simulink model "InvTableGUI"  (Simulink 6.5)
settings: Solver=FixedStepDiscrete  StartTime=0.0  StopTime=inf  FixedStep=samplePeriod  RelTol=1e-3
PreLoadFcn:
  | initialize
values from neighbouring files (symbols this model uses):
  accelCanon = 9810    [initialize.m]
  aInv = bFwd / bFwd(1)    [initialize.m]
  bInv = aFwd / bFwd(1)    [initialize.m]
  flowCanon = 1.666667e+04    (= 16666.67)    [initialize.m]    (also in Copy of initialize.m)
  forceCanon = 1    [initialize.m]    (also in Copy of initialize.m)
  friction = 5			 				* 0.155000	 				* 0.00444822 				* area1    (= 2.71252900422)    [initialize.m]
  gasConstant = 1.8    [initialize.m]    (also in Copy of initialize.m)
  iactParams = [actParams, dfGain, solver]    [initialize.m]
  lengthCanon = 1    [initialize.m]    (also in Copy of initialize.m)
  massCanon = 1e-06    [initialize.m]    (also in Copy of initialize.m)
  maxOilVolume = volume * (1 - (precharge/supplyPress)^(1/gasConstant))    (= 211.391477114)    [initialize.m]    (also in Copy of initialize.m)
  precharge = 3000		 				* 6.894757e-03    (= 20.684271)    [initialize.m]    (also in Copy of initialize.m)
  pumpFlow = 1e20    (= 1e+20)    [initialize.m]    (also in Copy of initialize.m)
  returnPress = 3			 				* 0.1    (= 0.3)    [initialize.m]    (also in Copy of initialize.m)
  rigidMass = 32900		 				+ (   3596	 				   +   528	 				   +    43	 				   +   122)	 				* 0.453592    (= 34845.456088)    [initialize.m]
  samplePeriod = controlPeriod/upsampleFactor    (= 0.0009765625)    [initialize.m]    (also in viewer.m = eval(getHeaderValue(header, 'DELTA_T')); Copy of initialize.m)
  supplyPress = 280		 				* 0.1    (= 28)    [initialize.m]    (also in Copy of initialize.m)
  velocCanon = 1    [initialize.m]    (also in Copy of initialize.m)
  volume = 15.15		 				+ (  45		 				    * 2		 				   + 30		 				    * 6 )	 				* 5    (= 1365.15)    [initialize.m]    (also in quake.m = volume / 231.0; Copy of initialize.m)
  volumeCanon = 1e+06    (= 1000000)    [initialize.m]    (also in Copy of initialize.m)
  yieldDispl = 1.0    (= 1)    [initialize.m]
undefined symbols (not defined in the file or in its folder): DiscIntNeverNeededParam
libraries: simulink x1

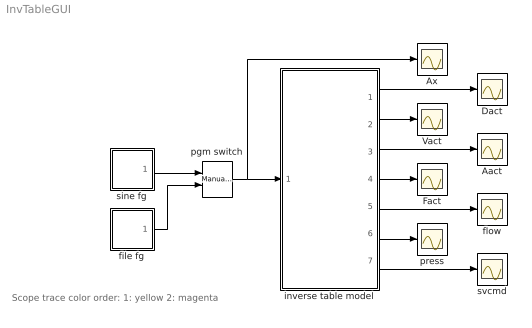
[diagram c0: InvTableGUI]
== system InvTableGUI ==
  note: Scope trace color order: 1: yellow 2: magenta
  Aact : Scope
  Ax : Scope
  Dact : Scope
  Fact : Scope
  Vact : Scope
  file fg : Subsystem
  flow : Scope
  inverse table model : Subsystem
  pgm switch : simulink/Signal Routing/Manual Switch  SystemSampleTime=-1  sw=1  action=0
  press : Scope
  sine fg : Subsystem  mask(Sine Function Generator){ampl=0.5, freq=0.5, spanInterval=1, samplePeriod=samplePeriod}
      mask prompts: ampl "Amplitude"; freq "Frequency (Hz)"; spanInterval "Span interval (sec)"; samplePeriod "Sample period (sec)"
  svcmd : Scope
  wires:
  sine fg/1(out) -> pgm switch/1
  pgm switch/1 -> Ax/1, inverse table model/1(Ax)
  inverse table model/1(Dact) -> Dact/1
  inverse table model/2(Vact) -> Vact/1
  inverse table model/3(Aact) -> Aact/1
  inverse table model/4(Fact) -> Fact/1
  inverse table model/5(flow) -> flow/1
  inverse table model/6(press) -> press/1
  inverse table model/7(svcmd) -> svcmd/1
  file fg/1(out) -> pgm switch/2

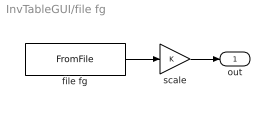
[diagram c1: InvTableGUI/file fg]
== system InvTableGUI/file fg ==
  file fg : FromFile  FileName=KobeAccel.mat  SampleTime=samplePeriod
  scale : Gain
  out : Outport
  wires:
  scale/1 -> out/1
  file fg/1 -> scale/1

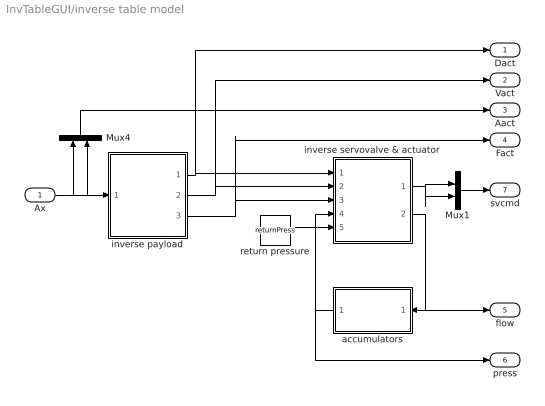
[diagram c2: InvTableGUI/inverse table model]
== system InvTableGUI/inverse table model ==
  Ax : Inport
  Mux1 : Mux  Inputs=2
  Mux4 : Mux  Orientation=up  Inputs=2
  accumulators : Subsystem  Orientation=left
  inverse payload : Subsystem
  inverse servovalve & actuator : Subsystem  mask(Inverse actuator){params=iactParams}
      mask prompts: params "Parameter vector"
  return pressure : Constant  Value=returnPress  OutDataType=sfix(16)  ConRadixGroup=Use specified scaling  OutScaling=2^0  SampleTime=inf  FramePeriod=inf
  Dact : Outport
  Vact : Outport  Port=2
  Aact : Outport  Port=3
  Fact : Outport  Port=4
  flow : Outport  Port=5
  press : Outport  Port=6
  svcmd : Outport  Port=7
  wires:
  inverse payload/3(force) -> inverse servovalve & actuator/3(force), Fact/1
  inverse payload/2(veloc) -> inverse servovalve & actuator/2(veloc), Vact/1
  inverse payload/1(displ) -> inverse servovalve & actuator/1(displ), Dact/1
  Mux1/1 -> svcmd/1
  inverse servovalve & actuator/1(cmd) -> Mux1/2, Mux1/1
  inverse servovalve & actuator/2(flow) -> flow/1, accumulators/1(flow)
  return pressure/1 -> inverse servovalve & actuator/5(rtn press)
  accumulators/1(press) -> inverse servovalve & actuator/4(spl press), press/1
  Mux4/1 -> Aact/1
  Ax/1 -> Mux4/2, inverse payload/1(accel), Mux4/1

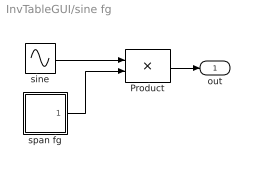
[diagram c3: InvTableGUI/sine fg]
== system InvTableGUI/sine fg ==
  Product : Product
  sine : Sin  Amplitude=ampl  Frequency=2 * pi * freq  SampleTime=samplePeriod
  span fg : Subsystem  mask{spanInterval=spanInterval, samplePeriod=samplePeriod}
      mask prompts: spanInterval "Span interval (sec)"; samplePeriod "Sample period (sec)"
  out : Outport
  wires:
  span fg/1(out) -> Product/2
  sine/1 -> Product/1
  Product/1 -> out/1

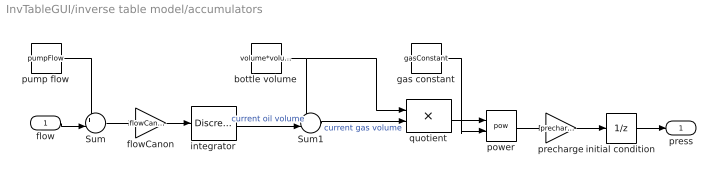
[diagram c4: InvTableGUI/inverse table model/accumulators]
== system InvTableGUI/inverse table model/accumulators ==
  flow : Inport
  Sum : Sum  Inputs=+-|
  Sum1 : Sum  Inputs=+-|
  bottle volume : Constant  Value=volume*volumeCanon  OutDataType=sfix(16)  ConRadixGroup=Use specified scaling  OutScaling=2^0  SampleTime=inf  FramePeriod=inf
  flowCanon : Gain  Gain=flowCanon
  gas constant : Constant  Value=gasConstant  OutDataType=sfix(16)  ConRadixGroup=Use specified scaling  OutScaling=2^0  SampleTime=inf  FramePeriod=inf
  initial condition : UnitDelay  X0=supplyPress  SampleTime=-1
  integrator : DiscreteIntegrator  InitialCondition=maxOilVolume*volumeCanon  SampleTime=-1  LimitOutput=on  UpperSaturationLimit=maxOilVolume*volumeCanon  LowerSaturationLimit=0  ICPrevOutput=DiscIntNeverNeededParam  ICPrevScaledInput=DiscIntNeverNeededParam
  power : Math  Operator=pow
  precharge : Gain  Gain=precharge
  pump flow : Constant  Value=pumpFlow  OutDataType=sfix(16)  ConRadixGroup=Use specified scaling  OutScaling=2^0  SampleTime=inf  FramePeriod=inf
  quotient : Product  Inputs=*/
  press : Outport
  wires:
  initial condition/1 -> press/1
  flowCanon/1 -> integrator/1
  flow/1 -> Sum/2
  integrator/1 -> Sum1/2  "current oil volume"
  quotient/1 -> power/1
  Sum1/1 -> quotient/2  "current gas volume"
  precharge/1 -> initial condition/1
  power/1 -> precharge/1
  gas constant/1 -> power/2
  bottle volume/1 -> quotient/1, Sum1/1
  Sum/1 -> flowCanon/1
  pump flow/1 -> Sum/1

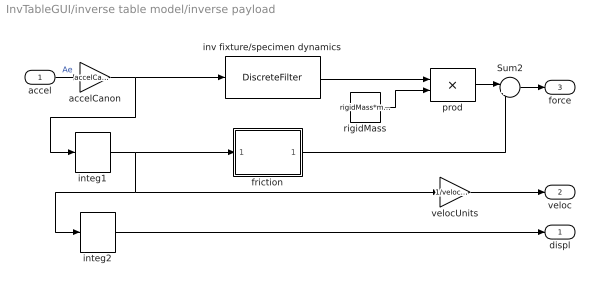
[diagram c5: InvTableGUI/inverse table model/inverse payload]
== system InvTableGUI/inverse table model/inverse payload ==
  accel : Inport
  Sum2 : Sum  Inputs=|++
  accelCanon : Gain  Gain=accelCanon
  friction : Subsystem  mask{friction=friction*forceCanon, yieldDispl=yieldDispl*lengthCanon, hysteresis=0}
      mask prompts: friction "Sliding friction"; yieldDispl "Equiv. yield displacement (in)"; hysteresis "Hysteresis constant"
  integ1 : DiscreteIntegrator  IntegratorMethod=Integration: Backward Euler  SampleTime=-1  ICPrevOutput=DiscIntNeverNeededParam  ICPrevScaledInput=DiscIntNeverNeededParam
  integ2 : DiscreteIntegrator  IntegratorMethod=Integration: Backward Euler  SampleTime=-1  ICPrevOutput=DiscIntNeverNeededParam  ICPrevScaledInput=DiscIntNeverNeededParam
  inv fixture/specimen dynamics : DiscreteFilter  Numerator=bInv  Denominator=aInv  SampleTime=-1
  prod : Product  Inputs=**
  rigidMass : Constant  Value=rigidMass*massCanon  OutDataType=sfix(16)  ConRadixGroup=Use specified scaling  OutScaling=2^0  SampleTime=inf  FramePeriod=inf
  velocUnits : Gain  Gain=1/velocCanon
  displ : Outport
  veloc : Outport  Port=2
  force : Outport  Port=3
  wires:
  velocUnits/1 -> veloc/1
  Sum2/1 -> force/1
  accel/1 -> accelCanon/1  "Ae"
  accelCanon/1 -> inv fixture/specimen dynamics/1, integ1/1
  integ1/1 -> velocUnits/1, integ2/1, friction/1(veloc)
  integ2/1 -> displ/1
  friction/1(force) -> Sum2/2
  inv fixture/specimen dynamics/1 -> prod/1
  prod/1 -> Sum2/1
  rigidMass/1 -> prod/2

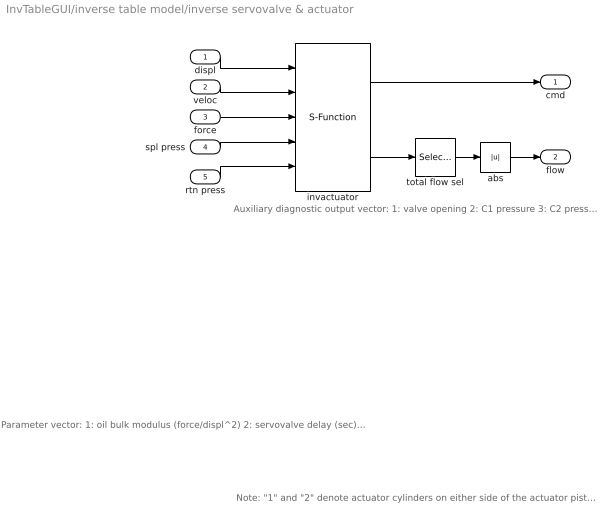
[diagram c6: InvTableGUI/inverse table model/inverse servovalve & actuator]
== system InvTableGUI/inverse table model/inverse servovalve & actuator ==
  note: Auxiliary diagnostic output vector: 1: valve opening 2: C1 pressure 3: C2 pressure 4: delta pressure 5: force 6: velocity 7: C1 flow 8: C2 flow 9: total flow 10: kinematic flow 11: compressibility flow 12: leakage flow 13: C1 oilspring displacement 14: C2 oilspring displacement 15: C1 oilspring velocity 16: C2 oilspring velocity 17: iteration error
  note: Note: "1" and "2" denote actuator cylinders on either side of the actuator piston. With positive valve drive, oil is ported into cylinder 1, resulting in positive displacement.
  note: Parameter vector: 1: oil bulk modulus (force/displ^2) 2: servovalve delay (sec) 3: servovalve overlap 4: rated pressure (force/displ^2) 5: rated flow at rated pressure (displ^3/sec) 6: nominal flow at rated pressure (displ^3/sec) 7: actuator piston area 1 (displ^2) 8: actuator piston area 2 (displ^2) 9: actuator usable stroke 1 (displ) 10: actuator usable stroke 2 (displ) 11: actuator end cushion length 1 (displ) 12: actuator end cushion length 2 (displ) 13: additional port volume 1 (displ^3) 14: additional port volume 1 (displ^3) 15: actuator parasitic damping factor 16: cross-chamber leakage factor (flow/press) 17: ratio port openings according to area 18: sample period (sec) Conversion factors used for converting signals from external (user) to internal (canonical) units: 19: displacement 20: velocity 21: force 22: pressure 23: flow Other: 24: delta-F feedback gain 25: inverse solver (0: exact, 1: approx)
  displ : Inport
  veloc : Inport  Port=2
  force : Inport  Port=3
  spl press : Inport  Port=4
  rtn press : Inport  Port=5
  abs : Abs  SaturateOnIntegerOverflow=on  SampleTime=-1
  invactuator : S-Function  FunctionName=InvActuator  Parameters=params
  total flow sel : Selector  InputType=Vector  ElementSrc=Internal  Elements=9  RowSrc=Internal  Rows=1  ColumnSrc=Internal  Columns=1  IndexIsStartValue=off
  cmd : Outport
  flow : Outport  Port=2
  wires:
  abs/1 -> flow/1
  total flow sel/1 -> abs/1
  invactuator/2 -> total flow sel/1
  force/1 -> invactuator/3
  veloc/1 -> invactuator/2
  invactuator/1 -> cmd/1
  displ/1 -> invactuator/1
  rtn press/1 -> invactuator/5
  spl press/1 -> invactuator/4

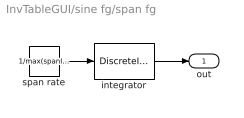
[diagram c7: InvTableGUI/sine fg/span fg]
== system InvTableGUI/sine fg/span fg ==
  integrator : DiscreteIntegrator  SampleTime=samplePeriod  LimitOutput=on  UpperSaturationLimit=1  LowerSaturationLimit=0  ICPrevOutput=DiscIntNeverNeededParam  ICPrevScaledInput=DiscIntNeverNeededParam
  span rate : Constant  Value=1/max(spanInterval,samplePeriod)  OutDataType=sfix(16)  ConRadixGroup=Use specified scaling  OutScaling=2^0  SampleTime=samplePeriod  FramePeriod=inf
  out : Outport
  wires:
  span rate/1 -> integrator/1
  integrator/1 -> out/1

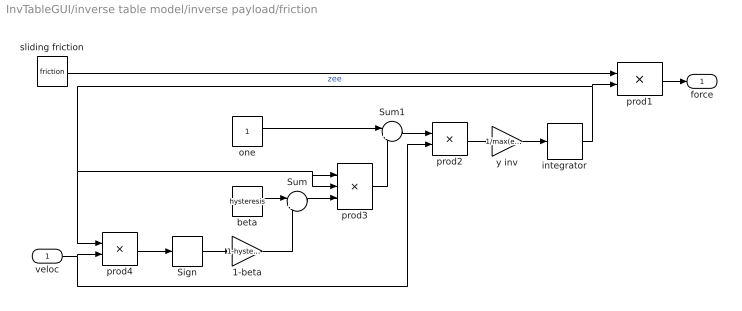
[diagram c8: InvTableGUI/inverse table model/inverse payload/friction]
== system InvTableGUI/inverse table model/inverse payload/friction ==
  veloc : Inport
  1-beta : Gain  Gain=1-hysteresis
  Sign : Signum
  Sum : Sum  Inputs=|++
  Sum1 : Sum  Inputs=|+-
  beta : Constant  Value=hysteresis  OutDataType=sfix(16)  ConRadixGroup=Use specified scaling  OutScaling=2^0  SampleTime=inf  FramePeriod=inf
  integrator : DiscreteIntegrator  SampleTime=-1  LimitOutput=on  UpperSaturationLimit=1  LowerSaturationLimit=-1  ICPrevOutput=DiscIntNeverNeededParam  ICPrevScaledInput=DiscIntNeverNeededParam
  one : Constant  Value=1  OutDataType=sfix(16)  ConRadixGroup=Use specified scaling  OutScaling=2^0  SampleTime=inf  FramePeriod=inf
  prod1 : Product
  prod2 : Product
  prod3 : Product  Inputs=3
  prod4 : Product
  sliding friction : Constant  Value=friction  OutDataType=sfix(16)  ConRadixGroup=Use specified scaling  OutScaling=2^0  SampleTime=inf  FramePeriod=inf
  y inv : Gain  Gain=1/max(eps, yieldDispl)
  force : Outport
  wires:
  sliding friction/1 -> prod1/1
  prod1/1 -> force/1
  veloc/1 -> prod4/2, prod2/2
  prod4/1 -> Sign/1
  Sign/1 -> 1-beta/1
  1-beta/1 -> Sum/2
  beta/1 -> Sum/1
  Sum/1 -> prod3/3
  one/1 -> Sum1/1
  prod3/1 -> Sum1/2
  Sum1/1 -> prod2/1
  prod2/1 -> y inv/1
  y inv/1 -> integrator/1
  integrator/1 -> prod1/2, prod4/1, prod3/1, prod3/2  "zee"
